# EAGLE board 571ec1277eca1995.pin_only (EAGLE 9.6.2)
REV: C

Size 85.72 x 53.98 mm. Coordinates in mm from the lower left corner, seen from the top.
Outline: 5.08,53.98 80.64,53.98 arc-90 85.72,48.9 85.72,5.08 arc-90 80.64,0 5.08,0 arc-90 0,5.08 0,48.9 arc-90 5.08,53.98
Copper layers (1*16): Top 0.035mm / dielectric 1.5mm / Bottom 0.035mm
Design rules "adafruit 7-7": minimum track width 7mil, minimum drill 15.5mil, track to track 7mil, track to pad 7mil, pad to pad 7mil, via to via 7mil, smd to smd 7mil, copper to edge 10mil, drill to drill 8mil, minimum pad ring 10mil, minimum via ring 8mil, stop-mask expansion 2mil, vias tented up to drill 20mil, thermal gap 10mil
Net classes: 3 Power: width 0.305 mm, drill 0.483 mm; 4 LOWPOWER: width 0.254 mm

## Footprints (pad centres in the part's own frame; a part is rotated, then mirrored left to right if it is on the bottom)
EVQ-Q2 = smd 3.2 x 1.2: A -3.4,-2; A' 3.4,-2; B -3.4,2; B' 3.4,2
0603-NO = smd 1.075 x 1: 1 -0.85,0; 2 0.85,0
0805-NO = smd 1.24 x 1.5: 1 -0.95,0; 2 0.95,0
0603-NO_WIDE = smd 0.9 x 1: 1 -0.85,0; 2 0.85,0
_1206 = smd 1.4 x 1.8: 1 -1.27,0; 2 1.27,0
JST_SH4 = smd 0.6 x 1.55: 1 -1.5,2.006; 2 -0.5,2.006; 3 0.5,2.006; 4 1.5,2.006 | smd 1.2 x 1.8: MT1 -2.8,-1.894; MT2 2.8,-1.894
SOD-323 = smd 1.35 x 0.8: A 1.27,0; C -1.27,0
JST_SH3_RA = smd 0.6 x 1.55: 1 1,0.924; 2 0,0.924; 3 -1,0.924 | smd 1.2 x 2.5: MT1 -2.3,-1.124; MT2 2.3,-1.124
1X01_ROUND = drill 1 pad 1.676: 1 0,0
SOT23-5L = smd 0.55 x 1.2: 1 -0.95,-1.3; 2 0,-1.3; 3 0.95,-1.3; 4 0.95,1.3; 5 -0.95,1.3
1X02_ROUND = drill 1 pad 1.778: 1 -1.27,0; 2 1.27,0
2X16 = drill 1.016 octagon: 1 -19.05,-1.27; 2 -19.05,1.27; 3 -16.51,-1.27; 4 -16.51,1.27; 5 -13.97,-1.27; 6 -13.97,1.27; 7 -11.43,-1.27; 8 -11.43,1.27; 9 -8.89,-1.27; 10 -8.89,1.27; 11 -6.35,-1.27; 12 -6.35,1.27; 13 -3.81,-1.27; 14 -3.81,1.27; 15 -1.27,-1.27; 16 -1.27,1.27; 17 1.27,-1.27; 18 1.27,1.27; 19 3.81,-1.27; 20 3.81,1.27; 21 6.35,-1.27; 22 6.35,1.27; 23 8.89,-1.27; 24 8.89,1.27; 25 11.43,-1.27; 26 11.43,1.27; 27 13.97,-1.27; 28 13.97,1.27; 29 16.51,-1.27; 30 16.51,1.27; 31 19.05,-1.27; 32 19.05,1.27
CHIPLED_0603_NOOUTLINE = smd 0.8 x 0.8: A 0,-0.75; C 0,0.75
INDUCTOR_1007 = smd 0.8 x 2: P$1 -1,0; P$2 1,0
LED3535_FULLPADS = smd 1 x 0.85: 1 -1.75,0.875 | smd 1.8 x 0.85: 2 -1.35,-0.875 | smd 1.2 x 0.85: 3 1.65,-0.875 | smd 2 x 0.85: 4 1.25,0.875
IRM-H6XXT = smd 0.7 x 1.4: 1 1.27,2.9; 2 -1.27,2.9; 3 -1.27,-2.9; 4 1.27,-2.9
SOT23-WIDE = smd 1 x 1.2: 1 -0.95,-1; 2 0.95,-1; 3 0,1
SOT363 = smd 0.5 x 0.5: 1 -0.75,-0.9; 3 0.75,-0.9; 4 0.75,0.9; 6 -0.75,0.9 | smd 0.4 x 0.5: 2 0,-0.9; 5 0,0.9
RESPACK_4X0603 = smd 0.45 x 0.9: 1 -1.3,-0.85; 2 -0.4,-0.85; 3 0.4,-0.85; 4 1.3,-0.85; 5 1.3,0.85; 6 0.4,0.85; 7 -0.4,0.85; 8 -1.3,0.85
JSTPH3 = smd 1 x 4.6: 1 -2,-2.7; 2 0,-2.7; 3 2,-2.7 | smd 1.6 x 3.4: NC1 -4.4,2.5; NC2 4.4,2.5
SOLDERJUMPER_2WAY_OPEN_NOPASTE = smd 1.168 x 1.6: 1 -1.397,0; 2 0,0; 3 1.397,0
SPDT_SS12D07VG5 = drill 1.2 pad 2: MNT1 4.15,0; MNT2 -4.15,0 | drill 0.8 pad 1.5: P 0,0; T1 -2,0; T2 2,0
TESTPOINT_ROUND_1.5MM_NO = smd 1.5 x 1.5: P$1 0,0
SMT_NUT_3MM = drill 4.25 pad 4.572: P$1 0,0
SOT23-DBV = smd 0.55 x 1.2: 1 -0.95,-1.3; 2 0,-1.3; 3 0.95,-1.3; 4 0.95,1.3; 5 -0.95,1.3
SOIC8_208MIL = smd 0.6 x 2.2: 1 -1.905,-3.315; 2 -0.635,-3.315; 3 0.635,-3.315; 4 1.905,-3.315; 5 1.905,3.315; 6 0.635,3.315; 7 -0.635,3.315; 8 -1.905,3.315
TLV320DAC3100 = smd 0.6 x 0.25: 1 -2.4,1.75; 2 -2.4,1.25; 3 -2.4,0.75; 4 -2.4,0.25; 5 -2.4,-0.25; 6 -2.4,-0.75; 7 -2.4,-1.25; 8 -2.4,-1.75; 17 2.4,-1.75; 18 2.4,-1.25; 19 2.4,-0.75; 20 2.4,-0.25; 21 2.4,0.25; 22 2.4,0.75; 23 2.4,1.25; 24 2.4,1.75 | smd 0.25 x 0.6: 9 -1.75,-2.4; 10 -1.25,-2.4; 11 -0.75,-2.4; 12 -0.25,-2.4; 13 0.25,-2.4; 14 0.75,-2.4; 15 1.25,-2.4; 16 1.75,-2.4; 25 1.75,2.4; 26 1.25,2.4; 27 0.75,2.4; 28 0.25,2.4; 29 -0.25,2.4; 30 -0.75,2.4; 31 -1.25,2.4; 32 -1.75,2.4 | smd 3.45 x 3.45: 33 0,0
SOT23-5 = smd 0.55 x 1.2: 1 -0.95,-1.3; 2 0,-1.3; 3 0.95,-1.3; 4 0.95,1.3; 5 -0.95,1.3
ESP32-PICO-MINI = smd 0.8 x 0.4: 1 -5.9,4; 2 -5.9,3.2; 3 -5.9,2.4; 4 -5.9,1.6; 5 -5.9,0.8; 6 -5.9,0; 7 -5.9,-0.8; 8 -5.9,-1.6; 9 -5.9,-2.4; 10 -5.9,-3.2; 11 -5.9,-4; 25 5.9,-4; 26 5.9,-3.2; 27 5.9,-2.4; 28 5.9,-1.6; 29 5.9,-0.8; 30 5.9,0; 31 5.9,0.8; 32 5.9,1.6; 33 5.9,2.4; 34 5.9,3.2; 35 5.9,4 | smd 0.4 x 0.8: 12 -4.8,-4.9; 13 -4,-4.9; 14 -3.2,-4.9; 15 -2.4,-4.9; 16 -1.6,-4.9; 17 -0.8,-4.9; 18 0,-4.9; 19 0.8,-4.9; 20 1.6,-4.9; 21 2.4,-4.9; 22 3.2,-4.9; 23 4,-4.9; 24 4.8,-4.9; 36 4.8,4.9; 37 4,4.9; 38 3.2,4.9; 39 2.4,4.9; 40 1.6,4.9; 41 0.8,4.9; 42 0,4.9; 43 -0.8,4.9; 44 -1.6,4.9; 45 -2.4,4.9; 46 -3.2,4.9; 47 -4,4.9; 48 -4.8,4.9 | smd 1.45 x 1.45: 49 0,0; 54 -1.95,0; 55 -1.95,-1.95; 56 0,-1.95; 57 1.95,-1.95; 58 1.95,0; 59 1.95,1.95; 60 0,1.95 | smd 0.7 x 0.7: 50 5.95,4.95; 51 5.95,-4.95; 52 -5.95,-4.95; 53 -5.95,4.95 | smd 0.5 x 0.5: 61 -1.95,1.95
MICROSD = smd 0.7 x 1.5: 1 1.761,-3.147; 2 0.661,-2.747; 3 -0.439,-3.147; 4 -1.539,-3.547; 5 -2.639,-3.147; 6 -3.739,-3.547; 7 -4.839,-3.147; 8 -5.939,-3.147 | smd 1.8 x 1.4: CD1 -5.239,7.053; CD2 0.38,7.053 | smd 1.4 x 1.9: MT1 -6.839,-6.047; MT2 6.361,-6.947
USB_TYPE_A_THM_SHORT = drill 0.95 long: D+ 1,1.5; D- -1,1.5; GND 3.5,1.5; VBUS -3.5,1.5 | drill 2 pad 3: S1 -6.4,0; S2 6.4,0
USB_C_CUSB31-CFM2AX-01-X = smd 0.575 x 1.15: A1B12 -3.2,2.275; A4B9 -2.4,2.275; B1A12 3.2,2.275; B4A9 2.4,2.275 | smd 0.275 x 1.15: A5 -1.25,2.275; A6 -0.25,2.275; A7 0.25,2.275; A8 1.25,2.275; B5 1.75,2.275; B6 0.75,2.275; B7 -0.75,2.275; B8 -1.75,2.275 | drill 0.6 pad 1 long: M1 -4.32,1.7; M2 4.32,1.7; M3 -4.32,-2.48; M4 4.32,-2.48 | hole 0.65: 2.89,1.2; -2.89,1.2
QFN80 = smd 0.78 x 0.22: 1 -5.09,3.8; 2 -5.09,3.4; 3 -5.09,3; 4 -5.09,2.6; 5 -5.09,2.2; 6 -5.09,1.8; 7 -5.09,1.4; 8 -5.09,1; 9 -5.09,0.6; 10 -5.09,0.2; 11 -5.09,-0.2; 12 -5.09,-0.6; 13 -5.09,-1; 14 -5.09,-1.4; 15 -5.09,-1.8; 16 -5.09,-2.2; 17 -5.09,-2.6; 18 -5.09,-3; 19 -5.09,-3.4; 20 -5.09,-3.8; 41 5.1,-3.8; 42 5.1,-3.4; 43 5.1,-3; 44 5.1,-2.6; 45 5.1,-2.2; 46 5.1,-1.8; 47 5.1,-1.4; 48 5.1,-1; 49 5.1,-0.6; 50 5.1,-0.2; 51 5.1,0.2; 52 5.1,0.6; 53 5.1,1; 54 5.1,1.4; 55 5.1,1.8; 56 5.1,2.2; 57 5.1,2.6; 58 5.1,3; 59 5.1,3.4; 60 5.1,3.8 | smd 0.22 x 0.78: 21 -3.8,-5.1; 22 -3.4,-5.1; 23 -3,-5.1; 24 -2.6,-5.1; 25 -2.2,-5.1; 26 -1.8,-5.1; 27 -1.4,-5.1; 28 -1,-5.1; 29 -0.6,-5.1; 30 -0.2,-5.1; 31 0.2,-5.1; 32 0.6,-5.1; 33 1,-5.1; 34 1.4,-5.1; 35 1.8,-5.1; 36 2.2,-5.1; 37 2.6,-5.1; 38 3,-5.1; 39 3.4,-5.1; 40 3.8,-5.1; 61 3.8,5.1; 62 3.4,5.1; 63 3,5.1; 64 2.6,5.1; 65 2.2,5.1; 66 1.8,5.1; 67 1.4,5.1; 68 1,5.1; 69 0.6,5.1; 70 0.2,5.1; 71 -0.2,5.1; 72 -0.6,5.1; 73 -1,5.1; 74 -1.4,5.1; 75 -1.8,5.1; 76 -2.2,5.1; 77 -2.6,5.1; 78 -3,5.1; 79 -3.4,5.1; 80 -3.8,5.1 | smd 3.4 x 3.4: MNT 0,0
QFN24_4MM = smd 0.8 x 0.28: 1 -2,1.25; 2 -2,0.75; 3 -2,0.25; 4 -2,-0.25; 5 -2,-0.75; 6 -2,-1.25; 13 2,-1.25; 14 2,-0.75; 15 2,-0.25; 16 2,0.25; 17 2,0.75; 18 2,1.25 | smd 0.28 x 0.8: 7 -1.25,-2; 8 -0.75,-2; 9 -0.25,-2; 10 0.25,-2; 11 0.75,-2; 12 1.25,-2; 19 1.25,2; 20 0.75,2; 21 0.25,2; 22 -0.25,2; 23 -0.75,2; 24 -1.25,2 | smd 1.778 x 1.778: THERM 0,0
HDMI_MOLEX_47151-0001 = smd 0.25 x 2.6: 1 4.5,3.302; 2 4,3.302; 3 3.5,3.302; 4 3,3.302; 5 2.5,3.302; 6 2,3.302; 7 1.5,3.302; 8 1,3.302; 9 0.5,3.302; 10 0,3.302; 11 -0.5,3.302; 12 -1,3.302; 13 -1.5,3.302; 14 -2,3.302; 15 -2.5,3.302; 16 -3,3.302; 17 -3.5,3.302; 18 -4,3.302; 19 -4.5,3.302 | drill 0.6 pad 1.65 long: P$1 -7.25,2.542; P$2 7.25,2.542 | drill 0.6 pad 1.5 long: P$3 7.25,-3.418; P$4 -7.25,-3.418
PJ-332A = drill 0.6 pad 1.651 long: 1 -4.792,-3; 2 -4.692,2.45 | smd 1.6 x 1.6: 3 -1.342,-3.65; 4 2.458,3.55; 5 4.158,-3.65; 6 4.658,3.55 | hole 1.4: -4.242,0; 2.758,0.1
53398-0271 = smd 0.8 x 1.6: 1 0.625,-1.27; 2 -0.625,-1.27 | smd 2.1 x 3: M1 3.185,1.48; M2 -3.185,1.48
CRYSTAL_2.5X2 = smd 0.9 x 0.75: 1 -0.825,-0.625; 2 0.825,-0.625; 3 0.825,0.625; 4 -0.825,0.625

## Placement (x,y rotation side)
BTN0  6MM_TACT  [EVQ-Q2]  80.45,11.43 0 top
BTN2  6MM_TACT  [EVQ-Q2]  80.45,27.94 0 top
BTN3  6MM_TACT  [EVQ-Q2]  80.45,19.56 0 top
C1  2.2uF  [0603-NO]  34.86,26.67 180 top
C2  1uF  [0603-NO]  51.75,34.61 45 top
C3  10uF  [0805-NO]  70.23,9.72 0 top
C4  2.2uF  [0603-NO]  37.66,23.3 270 top
C5  10uF  [0805-NO]  58.17,34.54 0 top
C6  0.1uF  [0603-NO]  32.66,23.34 270 top
C7  0.1uF  [0603-NO]  74.87,28.57 0 top
C8  0.1uF  [0603-NO]  54.17,30.1 180 top
C9  10uF  [0805-NO]  65.98,23.18 0 top
C10  10uF_0603  [0603-NO_WIDE]  39.93,23.99 180 top
C11  1uF  [0603-NO]  52.65,25.85 270 top
C12  1uF  [0603-NO]  32.26,32.32 180 top
C13  0.1uF  [0603-NO]  30.42,36.58 0 top
C14  0.1uF  [0603-NO]  40.89,40.13 0 top
C15  10uF_0603  [0603-NO_WIDE]  39.94,22.48 0 top
C16  1uF  [0603-NO]  54.17,31.62 0 top
C17  0.1uF  [0603-NO]  49.15,39.05 90 top
C18  10uF  [0805-NO]  57.98,28.64 180 top
C19  10uF  [0805-NO]  7.94,36.13 0 top
C20  10uF  [0805-NO]  36.39,19.75 0 top
C21  0.1uF  [0603-NO]  50.99,25.84 270 top
C22  0.1uF  [0603-NO]  42.29,21.27 270 top
C23  10uF  [0805-NO]  57.98,26.67 180 top
C24  0.1uF  [0603-NO]  46.86,39.81 0 top
C25  0.1uF  [0603-NO]  46.61,20.95 270 top
C26  15pF  [0603-NO]  48.2,41.34 180 top
C27  15pF  [0603-NO]  40.89,41.85 0 top
C28  1uF  [0603-NO]  51.37,18.1 0 top
C29  10uF  [0805-NO]  66.93,19.68 90 top
C30  1uF  [0603-NO]  65.09,19.81 90 top
C31  10uF  [0805-NO]  63.44,20.51 270 top
C32  100uF/6.3V  [_1206]  21.21,7.87 270 top
C33  0.1uF  [0603-NO]  32.26,30.8 0 top
C34  0.1uF  [0603-NO]  64.33,32.13 90 top
C35  0.1uF  [0603-NO]  77.91,34.04 180 top
C36  0.1uF  [0603-NO]  69.91,33.66 180 top
C37  0.1uF  [0603-NO]  61.79,27.11 180 top
C38  10uF  [0805-NO]  78.04,32.13 0 top
C39  0.1uF  [0603-NO]  70.23,8 180 top
C40  0.1uF  [0603-NO]  6.6,43.18 270 top
C41  10uF  [0805-NO]  74.1,25.34 270 top
C42  100uF/6.3V  [_1206]  73.85,34.23 0 top
C43  100uF/6.3V  [_1206]  72.39,40.77 90 top
C44  10uF  [0805-NO]  61.79,34.92 0 top
C45  10uF  [0805-NO]  61.79,28.89 180 top
C46  100uF/6.3V  [_1206]  68.58,5.08 270 top
C48  10uF  [0805-NO]  8,34.16 0 top
C50  10uF  [0805-NO]  5.71,45.72 180 top
C53  10uF  [0805-NO]  14.8,35.24 90 top
C54  10uF  [0805-NO]  2.16,45.72 0 top
C55  1uF  [0603-NO]  8,32.38 0 top
CONN1  STEMMA_I2C_QT  [JST_SH4]  72.96,3.11 0 top
D2  3.6V  [SOD-323]  11.37,14.92 90 top
D3  1N4148  [SOD-323]  49.09,19.68 270 top
DEBUG  JST_SH3  [JST_SH3_RA]  24,35.12 180 top
ESP_BOOT  [1X01_ROUND]  51.88,40.89 0 top
IC1  74AHC1G125  [SOT23-5L]  11.56,34.67 180 top
JP1  [1X02_ROUND]  70.74,13.46 270 top
JP3  2x16 SOCKET  [2X16]  42.86,9.53 180 top
L  RED  [CHIPLED_0603_NOOUTLINE]  36.98,51.05 180 top
L1  DFE252012F-3R3M=P2  [INDUCTOR_1007]  40.01,20.64 180 top
LED1  WS2812B_3535FULL  [LED3535_FULLPADS]  4,36 270 top
LED2  WS2812B_3535FULL  [LED3535_FULLPADS]  4,42.35 270 top
LED3  WS2812B_3535FULL  [LED3535_FULLPADS]  4,29.65 270 top
LED4  WS2812B_3535FULL  [LED3535_FULLPADS]  4,23.3 270 top
LED5  WS2812B_3535FULL  [LED3535_FULLPADS]  4,17.14 270 top
O1  GENERIC_IR_RECV_IRM-H6XXT  [IRM-H6XXT]  52.26,49.72 0 top
ON  GREEN  [CHIPLED_0603_NOOUTLINE]  48.79,50.8 0 top
P1LED  GREEN  [CHIPLED_0603_NOOUTLINE]  36.7,4.06 0 top
P2LED  GREEN  [CHIPLED_0603_NOOUTLINE]  49.02,4.06 180 top
PLABEL0  [PLABEL0]  49.02,52.83 0 top
PLABEL1  [PLABEL1]  36.96,53.02 0 top
PLABEL2  [PLABEL2]  73.79,47.18 0 top
PLABEL3  [PLABEL3]  16.26,15.88 0 top
PLABEL4  [PLABEL4]  80.64,23.94 0 top
PLABEL5  [PLABEL5]  80.84,15.56 0 top
PLABEL6  [PLABEL6]  80.58,7.56 0 top
PLABEL7  [PLABEL7]  77.34,1.33 90 top
PLABEL8  [PLABEL8]  5.21,7.68 0 top
PLABEL9  [PLABEL9]  23.75,13.21 90 top
PLABEL10  [PLABEL10]  26.29,13.14 90 top
PLABEL11  [PLABEL11]  28.83,12.83 0 top
PLABEL12  [PLABEL12]  31.69,12.89 0 top
PLABEL13  [PLABEL13]  34.04,12.89 0 top
PLABEL14  [PLABEL14]  36.58,12.89 0 top
PLABEL15  [PLABEL15]  39.18,12.83 0 top
PLABEL16  [PLABEL16]  41.66,12.83 0 top
PLABEL17  [PLABEL17]  44.26,12.83 0 top
PLABEL18  [PLABEL18]  46.86,12.83 0 top
PLABEL19  [PLABEL19]  49.28,12.83 0 top
PLABEL20  [PLABEL20]  51.82,12.89 0 top
PLABEL21  [PLABEL21]  53.98,12.89 0 top
PLABEL22  [PLABEL22]  56.83,12.83 0 top
PLABEL23  [PLABEL23]  59.63,12.83 0 top
PLABEL24  [PLABEL24]  62.1,12.83 0 top
PLABEL25  [PLABEL25]  45.85,0.95 0 top
PLABEL26  [PLABEL26]  39.94,0.95 0 top
PLABEL27  [PLABEL27]  22.99,16 0 top
PLABEL28  [PLABEL28]  21.27,24.7 0 top
PLABEL29  [PLABEL29]  23.24,32.64 0 top
PLABEL30  [PLABEL30]  63.56,43.12 0 top
PLABEL31  [PLABEL31]  76.14,11.49 90 top
PLABEL32  [PLABEL32]  1.02,29.46 90 top
PLABEL33  [PLABEL33]  7.24,1.4 90 top
PLABEL34  [PLABEL34]  53.47,45.34 0 top
PLABEL35  [PLABEL35]  29.02,53.21 0 top
PLABEL36  [PLABEL36]  0.95,27.24 0 bottom
PLABEL37  [PLABEL37]  63.75,21.65 0 bottom
PLABEL38  [PLABEL38]  15.88,1.21 90 bottom
PLABEL39  [PLABEL39]  9.65,1.21 90 bottom
PLABEL40  [PLABEL40]  14.99,3.49 0 bottom
PTC1  5V/1A  [0805-NO]  62.42,23.18 180 top
Q1  BSS138  [SOT23-WIDE]  55.18,22.29 0 top
Q2  BSS138 Dual  [SOT363]  64.96,40.51 0 top
Q3  DMP3098L  [SOT23-WIDE]  37.59,41.72 180 top
R1  10K  [0603-NO]  58.8,19.81 180 top
R2  10K  [0603-NO]  48.83,47.82 90 top
R3  10K  [0603-NO]  29.02,33.66 270 top
R4  220  [0603-NO]  34.23,23.37 270 top
R5  22 ohm  [0603-NO]  36.13,23.37 90 top
R6  10K  [0603-NO]  33.02,19.75 0 top
R7  10K  [0603-NO]  66.8,33.85 180 top
R8  10K  [0603-NO]  55.37,19.81 180 top
R9  5.1K  [0603-NO]  58.55,14.86 270 top
R10  10K  [0603-NO]  37.59,44.2 180 top
R11  2.2K  [0603-NO]  36.83,48.13 90 top
R12  220 Pack  [RESPACK_4X0603]  57.53,40.64 180 top
R13  10K  [0603-NO]  6.67,38.67 270 top
R14  220 Pack  [RESPACK_4X0603]  61.66,40.64 180 top
R15  10K Pack  [RESPACK_4X0603]  68.58,40.32 270 top
R16  100K  [0603-NO]  69.43,37.08 180 top
R17  10K  [0603-NO]  50.77,15.77 90 top
R18  100K  [0603-NO]  66.23,37.08 0 top
R19  5.1K  [0603-NO]  40.07,44.13 90 top
R20  5.1K  [0603-NO]  47.31,43.88 90 top
R21  10K  [0603-NO]  1.4,16.38 270 top
R22  2.2K  [0603-NO]  71.44,25.08 180 top
R23  1K  [0603-NO]  43.18,40.96 270 top
R24  22 ohm  [0603-NO]  44.26,45.28 0 top
R25  22 ohm  [0603-NO]  41.59,44.13 270 top
R26  1K  [0603-NO]  49.21,15.75 90 top
R27  10K  [0603-NO]  18.16,35.24 270 top
R28  2.2K  [0603-NO]  61.21,37.02 0 top
R32  10K  [0603-NO]  50.99,44.51 90 top
R38  1K  [0603-NO]  11.37,11.24 90 top
SENSE1  JST PH 3  [JSTPH3]  13.34,4.38 180 top
SJ1  [SOLDERJUMPER_2WAY_OPEN_NOPASTE]  13.34,2.1 180 bottom
SW1  6MM_TACT  [EVQ-Q2]  5.27,11.43 0 top
SW2  SS12D07VG5  [SPDT_SS12D07VG5]  42.86,4.32 180 top
T1  DMP3098L  [SOT23-WIDE]  58.8,22.35 0 top
TP1  [TESTPOINT_ROUND_1.5MM_NO]  80.64,10.16 0 bottom
TP2  DNP  [SMT_NUT_3MM]  3.81,50.16 0 top
TP3  SEWTAP_SMTNUTM3  [SMT_NUT_3MM]  81.92,50.16 0 top
TP4  SEWTAP_SMTNUTM3  [SMT_NUT_3MM]  81.92,3.81 0 top
TP5  SEWTAP_SMTNUTM3  [SMT_NUT_3MM]  3.81,3.81 0 top
U2  AP2112K-3.3  [SOT23-DBV]  57.85,31.69 180 top
U3  AP6404  [SOIC8_208MIL]  33.4,16.26 270 top
U4  TLV320DAC3100  [TLV320DAC3100]  70.17,28.89 0 top
U5  AP2127K-1.8  [SOT23-5]  61.79,31.88 180 top
U6  W25Q128  [SOIC8_208MIL]  43.24,16.07 90 top
U9  ESP32-C6-MINI_MINI  [ESP32-PICO-MINI]  14.1,42.67 0 top
U$72  [ADAFRUIT_5MM]  72.52,48.9 0 top
U$73  [SPEAKER_OVAL8OHM]  21.21,24.38 0 top
U$86  [STEMMAQT]  74.55,6.16 90 top
U$87  [PCBFEAT-REV-040]  8.51,24.32 0 top
U$114  [ADAFRUIT_TEXT_30MM]  79.88,29.08 0 bottom
X1  MICROSD  [MICROSD]  28.32,45.4 180 top
X2  USB_TYPEA  [USB_TYPE_A_THM_SHORT]  27.94,3.81 0 top
X3  USB Type C  [USB_C_CUSB31-CFM2AX-01-X]  42.86,49.97 180 top
X4  RP2350B  [QFN80]  42.86,30.61 180 top
X5  USB_TYPEA  [USB_TYPE_A_THM_SHORT]  57.78,3.81 0 top
X6  CH334F  [QFN24_4MM]  66.8,13.14 0 top
X7  47151-0001  [HDMI_MOLEX_47151-0001]  63.5,48.51 180 top
X8  TRRS_2SWITCH_PJ332A  [PJ-332A]  78.74,40.64 180 top
X9  CON_MOLEX_2P  [53398-0271]  17.21,11.11 0 top
Y1  12MHz_10pF_50ohm  [CRYSTAL_2.5X2]  45.34,42.16 90 top
Y2  12MHz  [CRYSTAL_2.5X2]  62.55,14.8 180 top

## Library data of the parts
BTN0 BTN2 BTN3 DEBUG SW1 X8 X9 = adafruit_electromech
C1-C46 C50 C53-C55 D2 D3 ESP_BOOT JP1 L1 PTC1 R1-R28 R32 R38 SJ1 TP1 U3 U4 U6 U$72 U$73 U$114 Y1 Y2 = microbuilder
C48 U$87 = microbuilder; REV: C
CONN1 = adafruit_electromech; LCSC: C2845363
IC1 = adafruit; ROT: 270
JP3 = pinhead; FORCETHM: 1
L ON P1LED P2LED Q1 Q3 T1 = microbuilder; ROT: 270
LED1-LED5 = microbuilder; ROT: 180
O1 = adafruit_sensor
PLABEL0 PLABEL1-PLABEL40 = pinguin
Q2 = microbuilder; JLC_ROTATION: 270
SENSE1 = adafruit_electromech; ROT: 180
SW2 TP2-TP5 X2 X5 = adafruit_electromech; FORCETHM: 1
U2 = SmartPrj
U5 = adafruit_power; JLC_ROTATION: 270
U9 = adafruit_wireless
U$86 = silks
X1 = adafruit_electromech; JLC_ROTATION: 90; LCSC: C125617
X3 = adafruit_electromech; LCSC: C165948
X4 = adafruit_micro
X6 = adafruit_micro; ROT: 270
X7 = adafruit_electromech; LCSC: C138388

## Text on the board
tNames: SCL | SDA | AREF | GND | 1 | ANALOG IN | IOREF | RESET | 3V3 | 5V | GND | VIN | A0 | A1 | A2 | A3 | A4 | A5
Pinguin_tBackup: MicroSD | L | ON | 23 | 22 | Stereo / Headphone | IR In | DVI Video | SWD Debug | #23 | NeoPixels | Fruit Jam / RP2350 / Mini Comp | Button #3 | RP2350 | 4-8Ω | Button #2 | 6- / 20V | Speaker | GND | 5V | 3V | GND | A1 | A2 | A3 | A4 | A5 | D6 | D7 | D9 | 10 | 3V | 5V | D8 | UF2 | Reset | Button #1 | DC | In | A0 | OFF | ON | I2C
Pinguin_bBackup: A RP2350-Based Microcomputer / Jam Packed with Hardware... / 16MB Flash+8MB PSRAM / DVI Video, 2x USB Host / I2S Speaker/Headphone / MicroSD Storage, IR Sensor / ESP32-C6 WiFi Co-Processor / 5x NeoPixels, 3x Buttons / On/Off Switch, GPIO Header / SWD Debug, Stemma QT I2C Port | JST / VCC | 3V | 5V
214bmp: D:/SmartProjects/Snc/a4_bn_logo2.bmp

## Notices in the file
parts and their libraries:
microbuilder: This work is placed in the public domain, and may be freely used for commercial and non-commercial work with the following conditions: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
